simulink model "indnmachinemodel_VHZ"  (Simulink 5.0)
settings: Solver=ode4  StartTime=0  StopTime=1.2  FixedStep=1e-6  MaxStep=10e-6  RelTol=1e-3  AbsTol=1e-6
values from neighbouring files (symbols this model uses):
  J = 0.0226    [PARAM.M]
  p = 4    [PARAM.M]
  Rr = .39    (= 0.39)    [PARAM.M]
  Rs = .19    (= 0.19)    [PARAM.M]
  Vd = 300    [PARAM.M]
  wb = 2*pi*fb    (= 628.318530718)    [PARAM.M]
  Xlr = wb*Llr    (= 0.376991118431)    [PARAM.M]
  Xls = wb*Lls    (= 0.131946891451)    [PARAM.M]
  Xmstar = 1/(1/Xls+1/Xm+1/Xlr)    (= 0.0940797800005)    [PARAM.M]
undefined symbols (not defined in the file or in its folder): magnitude
libraries: simulink x2

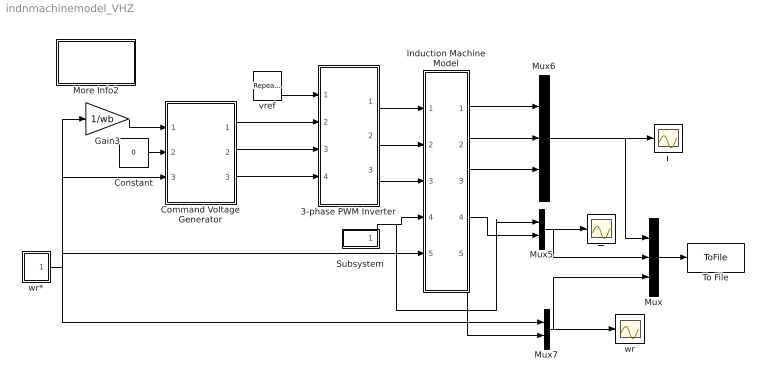
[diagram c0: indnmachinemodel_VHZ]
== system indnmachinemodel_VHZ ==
  3-phase PWM Inverter : Subsystem
  Command Voltage Generator : Subsystem
  Constant : Constant  Value=0
  Gain3 : Gain  Gain=1/wb
  Induction Machine Model : Subsystem
  More Info2 : Subsystem
  Mux : Mux  Inputs=3
  Mux5 : Mux  Inputs=2
  Mux6 : Mux  Inputs=3
  Mux7 : Mux  Inputs=2
  Subsystem : Subsystem
  T : Scope
  To File : ToFile  Filename=iemdc.mat  MatrixName=iemdc
  i : Scope
  vref : simulink/Sources/Repeating Sequence  rep_seq_t=[0 25e-6 50e-6 75e-6 100e-6]  rep_seq_y=[0 1 0 -1 0]
  wr : Scope
  wr* : Subsystem
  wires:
  Induction Machine Model/1(ia) -> Mux6/1
  Induction Machine Model/2(ib) -> Mux6/2
  Induction Machine Model/3(ic) -> Mux6/3
  Subsystem/1(Tl) -> Mux5/1, Induction Machine Model/4(Tl)
  Mux7/1 -> Mux/3, wr/1
  Mux5/1 -> Mux/2, T/1
  Induction Machine Model/4(Te) -> Mux5/2
  vref/1 -> 3-phase PWM Inverter/1(vref)
  wr*/1(wr*) -> Mux7/1, Induction Machine Model/5(we), Command Voltage Generator/3(we), Gain3/1
  Constant/1 -> Command Voltage Generator/2(vds*)
  Command Voltage Generator/1(vao*) -> 3-phase PWM Inverter/2(vao*)
  Command Voltage Generator/2(vbo*) -> 3-phase PWM Inverter/3(vbo*)
  Command Voltage Generator/3(vco*) -> 3-phase PWM Inverter/4(vco*)
  Induction Machine Model/5(wr) -> Mux7/2
  Gain3/1 -> Command Voltage Generator/1(vqs*)
  3-phase PWM Inverter/1(vao) -> Induction Machine Model/1(vao)
  3-phase PWM Inverter/2(vbo) -> Induction Machine Model/2(vbo)
  3-phase PWM Inverter/3(vco) -> Induction Machine Model/3(vco)
  Mux/1 -> To File/1
  Mux6/1 -> Mux/1, i/1

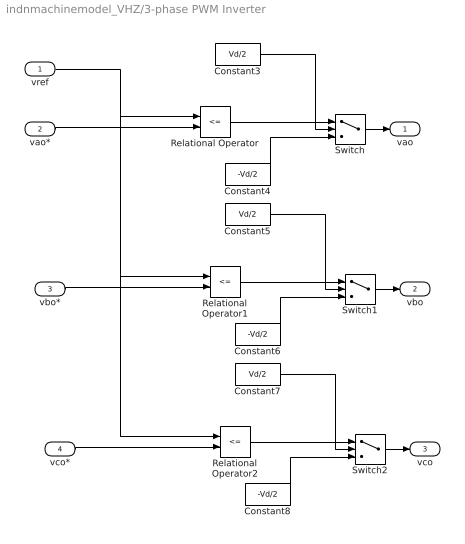
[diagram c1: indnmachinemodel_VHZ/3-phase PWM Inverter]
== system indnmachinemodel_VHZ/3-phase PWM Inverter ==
  vref : Inport
  vao* : Inport  Port=2
  vbo* : Inport  Port=3
  vco* : Inport  Port=4
  Constant3 : Constant  Value=Vd/2
  Constant4 : Constant  Value=-Vd/2
  Constant5 : Constant  Value=Vd/2
  Constant6 : Constant  Value=-Vd/2
  Constant7 : Constant  Value=Vd/2
  Constant8 : Constant  Value=-Vd/2
  Relational Operator : RelationalOperator  Operator=<=
  Relational Operator1 : RelationalOperator  Operator=<=
  Relational Operator2 : RelationalOperator  Operator=<=
  Switch : Switch  Threshold=0.5
  Switch1 : Switch  Threshold=0.5
  Switch2 : Switch  Threshold=0.5
  vao : Outport
  vbo : Outport  Port=2
  vco : Outport  Port=3
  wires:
  vao*/1 -> Relational Operator/2
  Switch/1 -> vao/1
  Constant4/1 -> Switch/3
  Constant3/1 -> Switch/1
  Relational Operator/1 -> Switch/2
  vbo*/1 -> Relational Operator1/2
  Switch1/1 -> vbo/1
  Constant6/1 -> Switch1/3
  Constant5/1 -> Switch1/1
  vco*/1 -> Relational Operator2/2
  Switch2/1 -> vco/1
  Constant8/1 -> Switch2/3
  Constant7/1 -> Switch2/1
  Relational Operator2/1 -> Switch2/2
  vref/1 -> Relational Operator/1, Relational Operator1/1, Relational Operator2/1
  Relational Operator1/1 -> Switch1/2

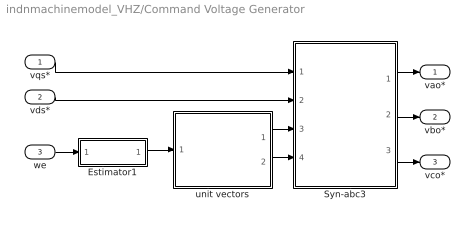
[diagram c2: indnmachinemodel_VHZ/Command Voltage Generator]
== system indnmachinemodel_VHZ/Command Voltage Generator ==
  vqs* : Inport
  vds* : Inport  Port=2
  we : Inport  Port=3
  Estimator1 : Subsystem
  Syn-abc3 : Subsystem
  unit vectors : Subsystem
  vao* : Outport
  vbo* : Outport  Port=2
  vco* : Outport  Port=3
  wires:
  Syn-abc3/1(vao*) -> vao*/1
  unit vectors/1(cos(theta-e)) -> Syn-abc3/3(cos(theta-e))
  unit vectors/2(sin(theta-e)) -> Syn-abc3/4(sin(theta-e))
  Estimator1/1(theta-e) -> unit vectors/1(theta-e)
  we/1 -> Estimator1/1(we)
  vds*/1 -> Syn-abc3/2(vds)
  vqs*/1 -> Syn-abc3/1(vqs)
  Syn-abc3/2(vbo*) -> vbo*/1
  Syn-abc3/3(vco*) -> vco*/1

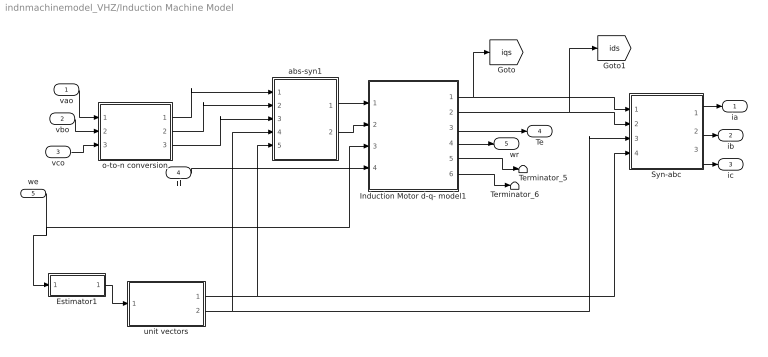
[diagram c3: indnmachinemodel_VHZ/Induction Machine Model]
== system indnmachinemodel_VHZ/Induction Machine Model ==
  vao : Inport
  vbo : Inport  Port=2
  vco : Inport  Port=3
  Tl : Inport  Port=4
  we : Inport  Port=5
  Estimator1 : Subsystem
  Induction Motor d-q- model1 : Subsystem
  Syn-abc : Subsystem
  Terminator_5 : Terminator
  Terminator_6 : Terminator
  abs-syn1 : Subsystem
  o-to-n conversion : Subsystem
  unit vectors : Subsystem
  ia : Outport
  ib : Outport  Port=2
  ic : Outport  Port=3
  Te : Outport  Port=4
  wr : Outport  Port=5
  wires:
  we/1 -> Induction Motor d-q- model1/3(we), Estimator1/1(we)
  Estimator1/1(theta-e) -> unit vectors/1(theta-e)
  Induction Motor d-q- model1/6("iqr ") -> Terminator_6/1
  Tl/1 -> Induction Motor d-q- model1/4(Tl)
  Syn-abc/2(ib) -> ib/1
  Syn-abc/3(ic) -> ic/1
  Induction Motor d-q- model1/5("idr ") -> Terminator_5/1
  Syn-abc/1(ia) -> ia/1
  Induction Motor d-q- model1/3("Te ") -> Te/1
  Induction Motor d-q- model1/4("wr ") -> wr/1
  vao/1 -> o-to-n conversion/1(vao)
  vbo/1 -> o-to-n conversion/2(vbo)
  vco/1 -> o-to-n conversion/3(vco)
  unit vectors/1(sin(theta-e)) -> Syn-abc/4(sin(theta-e)), abs-syn1/5(sin(theta-e))
  unit vectors/2(cos(theta-e)) -> Syn-abc/3(cos(theta-e)), abs-syn1/4(cos(theta-e))
  Induction Motor d-q- model1/2("ids ") -> Syn-abc/2(ids), [ids]
  Induction Motor d-q- model1/1("iqs ") -> [iqs], Syn-abc/1(iqs)
  o-to-n conversion/1(van) -> abs-syn1/1(van)
  o-to-n conversion/2(vbn) -> abs-syn1/2(vbn)
  o-to-n conversion/3(vcn) -> abs-syn1/3(vcn)
  abs-syn1/2(vds) -> Induction Motor d-q- model1/2(vds)
  abs-syn1/1(vqs) -> Induction Motor d-q- model1/1(vqs)

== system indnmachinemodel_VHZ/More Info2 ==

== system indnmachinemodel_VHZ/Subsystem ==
  Step2 : Step  Time=.8  After=20  SampleTime=0
  Step3 : Step  After=-10  SampleTime=0
  Step4 : Step  Time=30  After=0  SampleTime=0
  Sum1 : Sum  Inputs=|+++
  Tl : Outport
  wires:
  Step3/1 -> Sum1/2
  Step2/1 -> Sum1/1
  Step4/1 -> Sum1/3
  Sum1/1 -> Tl/1

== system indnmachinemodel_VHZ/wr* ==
  Gain2 : Gain
  Repeating Sequence : simulink/Sources/Repeating Sequence  rep_seq_t=[0 .15 .35 .4 .55 .6 10]  rep_seq_y=[0 .8*wb .8*wb .50*wb .50*wb .65*wb .65*wb]
  Saturation1 : Saturate  UpperLimit=.75*wb  LowerLimit=-.75*wb
  wr* : Outport
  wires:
  Repeating Sequence/1 -> Saturation1/1
  Saturation1/1 -> Gain2/1
  Gain2/1 -> wr*/1

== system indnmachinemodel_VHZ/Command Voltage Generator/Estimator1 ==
  we : Inport
  Constant : Constant  Value=2*pi
  Integrator : Integrator
  Math Function3 : Math  Operator=mod
  theta-e : Outport
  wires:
  Math Function3/1 -> theta-e/1
  Integrator/1 -> Math Function3/1
  Constant/1 -> Math Function3/2
  we/1 -> Integrator/1

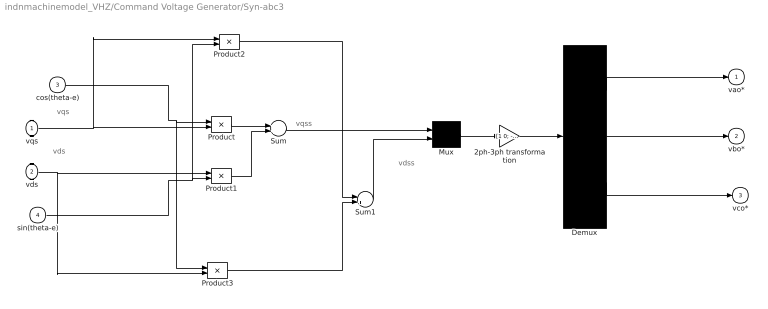
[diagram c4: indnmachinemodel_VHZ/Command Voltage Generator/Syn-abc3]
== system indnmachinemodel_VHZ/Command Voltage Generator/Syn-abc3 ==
  note: vqss
  note: vqs
  note: vdss
  note: vds
  vqs : Inport
  vds : Inport  Port=2
  cos(theta-e) : Inport  Port=3
  sin(theta-e) : Inport  Port=4
  2ph-3ph transformation : Gain  Gain="[1 0; -1/2 -sqrt(3)/2;  -1/2 sqrt(3)/2]"  Multiplication=Matrix(K*u)
  Demux : Demux  Outputs=3
  Mux : Mux  Inputs=2
  Product{,1..3} (4 alike) : Product
  Sum : Sum
  Sum1 : Sum  Inputs=-+
  vao* : Outport
  vbo* : Outport  Port=2
  vco* : Outport  Port=3
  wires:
  2ph-3ph transformation/1 -> Demux/1
  Sum1/1 -> Mux/2
  Product/1 -> Sum/1
  Product1/1 -> Sum/2
  sin(theta-e)/1 -> Product2/2, Product1/2
  cos(theta-e)/1 -> Product3/1, Product/1
  Product3/1 -> Sum1/2
  Product2/1 -> Sum1/1
  Mux/1 -> 2ph-3ph transformation/1
  vds/1 -> Product3/2, Product1/1
  vqs/1 -> Product2/1, Product/2
  Demux/1 -> vao*/1
  Demux/2 -> vbo*/1
  Demux/3 -> vco*/1
  Sum/1 -> Mux/1

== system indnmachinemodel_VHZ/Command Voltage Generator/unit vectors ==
  theta-e : Inport
  Trigonometric Function : Trigonometry
  Trigonometric Function1 : Trigonometry  Operator=cos
  cos(theta-e) : Outport
  sin(theta-e) : Outport  Port=2
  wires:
  Trigonometric Function/1 -> sin(theta-e)/1
  Trigonometric Function1/1 -> cos(theta-e)/1
  theta-e/1 -> Trigonometric Function1/1, Trigonometric Function/1

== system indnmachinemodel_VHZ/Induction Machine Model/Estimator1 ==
  we : Inport
  Constant : Constant  Value=2*pi
  Integrator : Integrator  InitialCondition=0.01
  Math Function3 : Math  Operator=mod
  theta-e : Outport
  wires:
  we/1 -> Integrator/1
  Constant/1 -> Math Function3/2
  Integrator/1 -> Math Function3/1
  Math Function3/1 -> theta-e/1

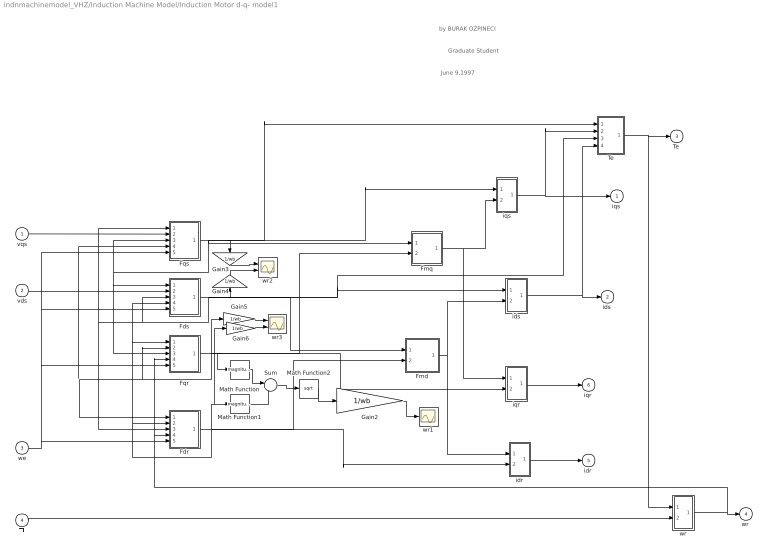
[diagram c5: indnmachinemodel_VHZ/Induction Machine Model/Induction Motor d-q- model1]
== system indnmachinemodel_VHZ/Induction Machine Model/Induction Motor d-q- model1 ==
  note: by BURAK OZPINECI
  note: Graduate Student
  note: June 9,1997
  vqs : Inport
  vds : Inport  Port=2
  we : Inport  Port=3
  Tl : Inport  Port=4
  Fdr : Subsystem
  Fds : Subsystem
  Fmd : Subsystem
  Fmq : Subsystem
  Fqr : Subsystem
  Fqs : Subsystem
  Gain2 : Gain  Gain=1/wb
  Gain3 : Gain  Orientation=down  Gain=1/wb
  Gain4 : Gain  Orientation=up  Gain=1/wb
  Gain5 : Gain  Gain=1/wb
  Gain6 : Gain  Gain=1/wb
  Math Function : Math  Operator=magnitude^2
  Math Function1 : Math  Operator=magnitude^2
  Math Function2 : Math  Operator=sqrt
  Sum : Sum  Inputs=|++
  Te : Subsystem
  idr : Subsystem
  ids : Subsystem
  iqr : Subsystem
  iqs : Subsystem
  wr : Subsystem
  wr1 : Scope
  wr2 : Scope  NumInputPorts=2
  wr3 : Scope  NumInputPorts=2
  "iqs " : Outport
  "ids " : Outport  Port=2
  "Te " : Outport  Port=3
  "wr " : Outport  Port=4
  "idr " : Outport  Port=5
  "iqr " : Outport  Port=6
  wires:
  Fdr/1("Fdr ") -> idr/2(Fdr), Fdr/2(Fdr), Fqr/1(Fdr), Fds/4(Fdr), Fmd/2(Fdr), Math Function1/1, Gain6/1
  we/1 -> Fqs/5(we), Fds/5(we), Fqr/5(we), Fdr/5(we)
  wr/1(wr) -> "wr "/1, Fqr/4(wr), Fdr/4(wr)
  vqs/1 -> Fqs/2(Vqs)
  vds/1 -> Fds/2(Vds)
  Tl/1 -> wr/2(Tl)
  Fqs/1("Fqs ") -> Fqs/3(Fqs), Fqr/3(Fqs), Fds/1(Fqs), Fmq/1(Fqs), iqs/1(Fqs), Te/1(Fqs), Gain3/1
  Fqr/1("Fqr ") -> Fqr/2(Fqr), Fqs/4(Fqr), Fdr/1(Fqr), Fmq/2(Fqr), Math Function/1, iqr/2(Fqr), Gain5/1
  Fds/1("Fds ") -> Fds/3(Fds), Fqs/1(Fds), Fdr/3(Fds), Fmd/1(Fds), ids/1(Fds), Te/3(Fds), Gain4/1
  iqr/1(iqr) -> "iqr "/1
  Fmq/1(Fmq) -> iqs/2(Fmq), iqr/1(Fmq)
  idr/1(idr) -> "idr "/1
  Fmd/1(Fmd) -> ids/2(Fmd), idr/1(Fmd)
  Te/1(Te) -> "Te "/1, wr/1(Te)
  ids/1(ids) -> "ids "/1, Te/4(ids)
  iqs/1(iqs) -> "iqs "/1, Te/2(iqs)
  Math Function/1 -> Sum/1
  Math Function1/1 -> Sum/2
  Sum/1 -> Math Function2/1
  Math Function2/1 -> Gain2/1
  Gain2/1 -> wr1/1
  Gain3/1 -> wr2/1
  Gain4/1 -> wr2/2
  Gain5/1 -> wr3/1
  Gain6/1 -> wr3/2

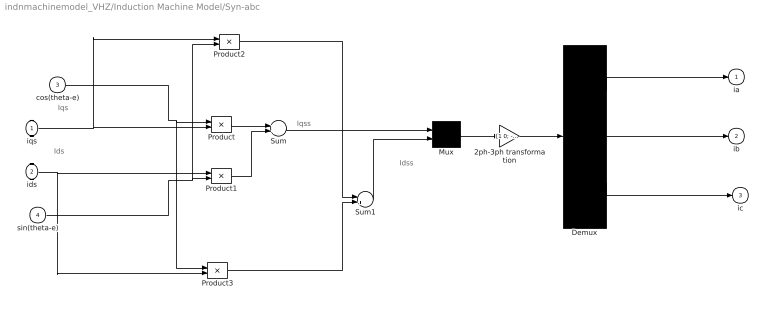
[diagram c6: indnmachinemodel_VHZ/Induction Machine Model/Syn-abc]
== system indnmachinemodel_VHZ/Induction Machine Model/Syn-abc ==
  note: Iqss
  note: Iqs
  note: Idss
  note: Ids
  iqs : Inport
  ids : Inport  Port=2
  cos(theta-e) : Inport  Port=3
  sin(theta-e) : Inport  Port=4
  2ph-3ph transformation : Gain  Gain="[1 0; -1/2 -sqrt(3)/2;  -1/2 sqrt(3)/2]"  Multiplication=Matrix(K*u)
  Demux : Demux  Outputs=3
  Mux : Mux  Inputs=2
  Product{,1..3} (4 alike) : Product
  Sum : Sum
  Sum1 : Sum  Inputs=-+
  ia : Outport
  ib : Outport  Port=2
  ic : Outport  Port=3
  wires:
  2ph-3ph transformation/1 -> Demux/1
  Sum1/1 -> Mux/2
  Sum/1 -> Mux/1
  Product/1 -> Sum/1
  Product1/1 -> Sum/2
  sin(theta-e)/1 -> Product2/2, Product1/2
  cos(theta-e)/1 -> Product3/1, Product/1
  Product3/1 -> Sum1/2
  Product2/1 -> Sum1/1
  Mux/1 -> 2ph-3ph transformation/1
  ids/1 -> Product3/2, Product1/1
  iqs/1 -> Product2/1, Product/2
  Demux/1 -> ia/1
  Demux/2 -> ib/1
  Demux/3 -> ic/1

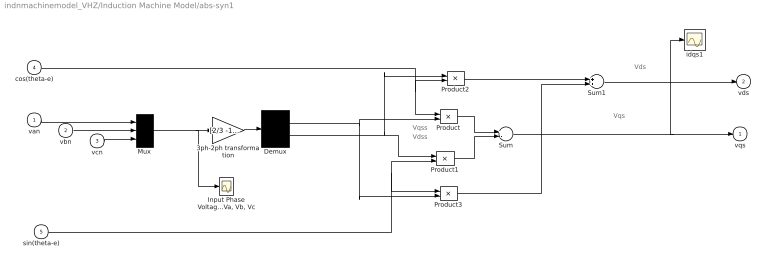
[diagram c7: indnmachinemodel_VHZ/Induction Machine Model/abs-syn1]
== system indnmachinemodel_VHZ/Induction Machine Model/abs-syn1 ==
  note: Vqs
  note: Vds
  note: Vqss
  note: Vdss
  van : Inport
  vbn : Inport  Port=2
  vcn : Inport  Port=3
  cos(theta-e) : Inport  Port=4
  sin(theta-e) : Inport  Port=5
  3ph-2ph transformation : Gain  Gain=[2/3 -1/3 -1/3;0 -1/sqrt(3) 1/sqrt(3)]  Multiplication=Matrix(K*u)
  Demux : Demux  Outputs=2
  "Input Phase Voltages Va, Vb, Vc" : Scope
  Mux : Mux  Inputs=3
  Product{,1..3} (4 alike) : Product
  Sum : Sum  Inputs=+-
  Sum1 : Sum
  idqs1 : Scope
  vqs : Outport
  vds : Outport  Port=2
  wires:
  cos(theta-e)/1 -> Product2/2, Product/1
  sin(theta-e)/1 -> Product3/1, Product1/2
  Demux/1 -> Product3/2, Product/2
  van/1 -> Mux/1
  Demux/2 -> Product1/1, Product2/1
  vbn/1 -> Mux/2
  Product3/1 -> Sum1/2
  Product2/1 -> Sum1/1
  Sum/1 -> idqs1/1, vqs/1
  Sum1/1 -> vds/1
  Product1/1 -> Sum/2
  Mux/1 -> 3ph-2ph transformation/1, "Input Phase Voltages Va, Vb, Vc"/1
  vcn/1 -> Mux/3
  Product/1 -> Sum/1
  3ph-2ph transformation/1 -> Demux/1

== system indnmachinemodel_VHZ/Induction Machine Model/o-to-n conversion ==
  vao : Inport
  vbo : Inport  Port=2
  vco : Inport  Port=3
  Demux : Demux  Outputs=3
  Matrix Gain : Gain  Gain=[2/3 -1/3 -1/3; -1/3 2/3 -1/3; -1/3 -1/3 2/3]  Multiplication=Matrix(K*u)
  Mux : Mux  Inputs=3
  van : Outport
  vbn : Outport  Port=2
  vcn : Outport  Port=3
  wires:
  Demux/3 -> vcn/1
  Demux/2 -> vbn/1
  Demux/1 -> van/1
  vco/1 -> Mux/3
  vbo/1 -> Mux/2
  vao/1 -> Mux/1
  Matrix Gain/1 -> Demux/1
  Mux/1 -> Matrix Gain/1

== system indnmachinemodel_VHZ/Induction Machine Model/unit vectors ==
  theta-e : Inport
  Trigonometric Function : Trigonometry
  Trigonometric Function1 : Trigonometry  Operator=cos
  sin(theta-e) : Outport
  cos(theta-e) : Outport  Port=2
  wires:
  theta-e/1 -> Trigonometric Function/1, Trigonometric Function1/1
  Trigonometric Function1/1 -> cos(theta-e)/1
  Trigonometric Function/1 -> sin(theta-e)/1

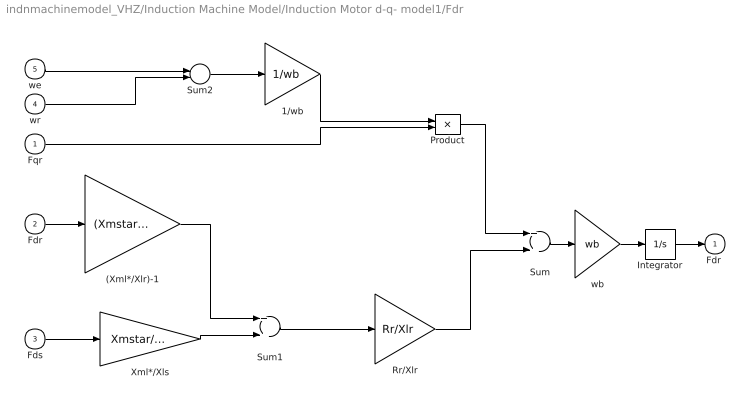
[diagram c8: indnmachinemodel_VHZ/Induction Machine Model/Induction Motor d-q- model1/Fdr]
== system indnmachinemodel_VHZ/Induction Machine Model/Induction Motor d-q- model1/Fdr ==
  Fqr : Inport
  Fdr : Inport  Port=2
  Fds : Inport  Port=3
  wr : Inport  Port=4
  we : Inport  Port=5
  (Xml*/Xlr)-1 : Gain  Gain=(Xmstar/Xlr)-1
  1/wb : Gain  Gain=1/wb
  Integrator : Integrator
  Product : Product
  Rr/Xlr : Gain  Gain=Rr/Xlr
  Sum : Sum
  Sum1 : Sum
  Sum2 : Sum  Inputs=+-
  Xml*/Xls : Gain  Gain=Xmstar/Xls
  wb : Gain  Gain=wb
  "Fdr " : Outport
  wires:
  Rr/Xlr/1 -> Sum/2
  Xml*/Xls/1 -> Sum1/2
  (Xml*/Xlr)-1/1 -> Sum1/1
  Product/1 -> Sum/1
  1/wb/1 -> Product/1
  wr/1 -> Sum2/2
  Fqr/1 -> Product/2
  we/1 -> Sum2/1
  Sum2/1 -> 1/wb/1
  Fds/1 -> Xml*/Xls/1
  Integrator/1 -> "Fdr "/1
  Fdr/1 -> (Xml*/Xlr)-1/1
  Sum1/1 -> Rr/Xlr/1
  Sum/1 -> wb/1
  wb/1 -> Integrator/1

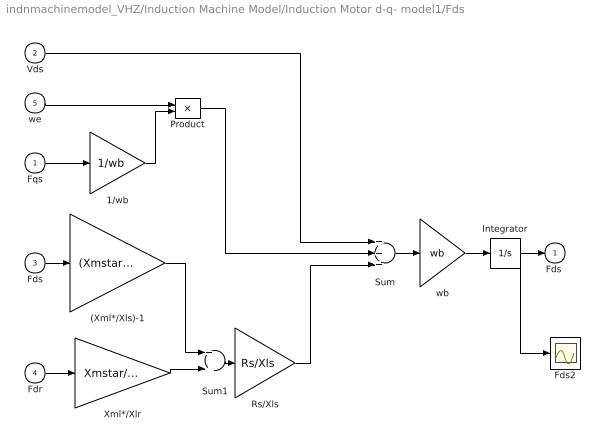
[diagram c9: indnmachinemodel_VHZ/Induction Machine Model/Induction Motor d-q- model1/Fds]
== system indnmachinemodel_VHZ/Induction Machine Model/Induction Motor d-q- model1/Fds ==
  Fqs : Inport
  Vds : Inport  Port=2
  Fds : Inport  Port=3
  Fdr : Inport  Port=4
  we : Inport  Port=5
  (Xml*/Xls)-1 : Gain  Gain=(Xmstar/Xls)-1
  1/wb : Gain  Gain=1/wb
  Fds2 : Scope
  Integrator : Integrator
  Product : Product
  Rs/Xls : Gain  Gain=Rs/Xls
  Sum : Sum  Inputs=+++
  Sum1 : Sum
  Xml*/Xlr : Gain  Gain=Xmstar/Xlr
  wb : Gain  Gain=wb
  "Fds " : Outport
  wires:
  1/wb/1 -> Product/2
  Product/1 -> Sum/2
  we/1 -> Product/1
  wb/1 -> Integrator/1
  Fdr/1 -> Xml*/Xlr/1
  Fds/1 -> (Xml*/Xls)-1/1
  Vds/1 -> Sum/1
  Fqs/1 -> 1/wb/1
  Rs/Xls/1 -> Sum/3
  (Xml*/Xls)-1/1 -> Sum1/1
  Xml*/Xlr/1 -> Sum1/2
  Sum1/1 -> Rs/Xls/1
  Sum/1 -> wb/1
  Integrator/1 -> "Fds "/1, Fds2/1

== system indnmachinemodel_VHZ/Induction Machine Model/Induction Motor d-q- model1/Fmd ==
  Fds : Inport
  Fdr : Inport  Port=2
  Sum8 : Sum
  Xmstar/Xlr : Gain  Gain=Xmstar/Xlr
  Xmstar/Xls : Gain  Gain=Xmstar/Xls
  Fmd : Outport
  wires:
  Fdr/1 -> Xmstar/Xlr/1
  Sum8/1 -> Fmd/1
  Fds/1 -> Xmstar/Xls/1
  Xmstar/Xls/1 -> Sum8/1
  Xmstar/Xlr/1 -> Sum8/2

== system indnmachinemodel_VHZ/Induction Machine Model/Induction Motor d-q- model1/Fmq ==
  Fqs : Inport
  Fqr : Inport  Port=2
  Sum8 : Sum
  Xmstar/Xlr : Gain  Gain=Xmstar/Xlr
  Xmstar/Xls : Gain  Gain=Xmstar/Xls
  Fmq : Outport
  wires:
  Fqr/1 -> Xmstar/Xlr/1
  Sum8/1 -> Fmq/1
  Fqs/1 -> Xmstar/Xls/1
  Xmstar/Xls/1 -> Sum8/1
  Xmstar/Xlr/1 -> Sum8/2

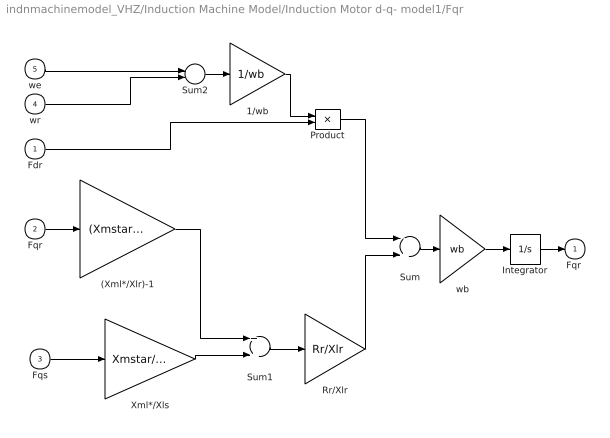
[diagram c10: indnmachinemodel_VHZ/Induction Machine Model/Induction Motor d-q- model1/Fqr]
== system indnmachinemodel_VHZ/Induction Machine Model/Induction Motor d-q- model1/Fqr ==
  Fdr : Inport
  Fqr : Inport  Port=2
  Fqs : Inport  Port=3
  wr : Inport  Port=4
  we : Inport  Port=5
  (Xml*/Xlr)-1 : Gain  Gain=(Xmstar/Xlr)-1
  1/wb : Gain  Gain=1/wb
  Integrator : Integrator
  Product : Product
  Rr/Xlr : Gain  Gain=Rr/Xlr
  Sum : Sum  Inputs=-+
  Sum1 : Sum
  Sum2 : Sum  Inputs=+-
  Xml*/Xls : Gain  Gain=Xmstar/Xls
  wb : Gain  Gain=wb
  "Fqr " : Outport
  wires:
  (Xml*/Xlr)-1/1 -> Sum1/1
  Rr/Xlr/1 -> Sum/2
  Product/1 -> Sum/1
  Fdr/1 -> Product/2
  1/wb/1 -> Product/1
  Sum2/1 -> 1/wb/1
  wr/1 -> Sum2/2
  we/1 -> Sum2/1
  Fqs/1 -> Xml*/Xls/1
  Integrator/1 -> "Fqr "/1
  Fqr/1 -> (Xml*/Xlr)-1/1
  Xml*/Xls/1 -> Sum1/2
  Sum1/1 -> Rr/Xlr/1
  Sum/1 -> wb/1
  wb/1 -> Integrator/1

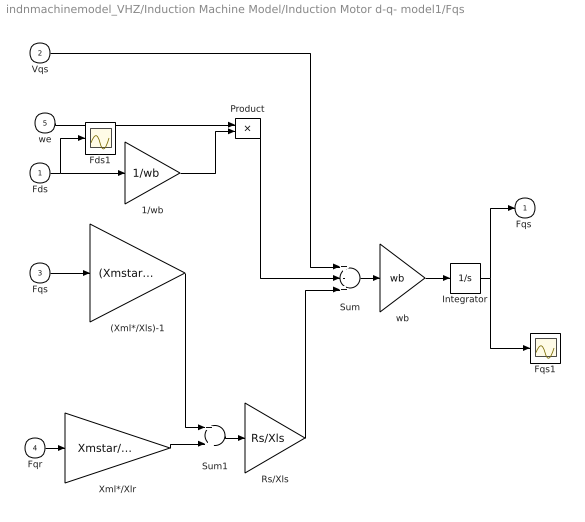
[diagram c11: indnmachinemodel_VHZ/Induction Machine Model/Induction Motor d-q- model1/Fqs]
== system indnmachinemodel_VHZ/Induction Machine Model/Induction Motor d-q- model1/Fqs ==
  Fds : Inport
  Vqs : Inport  Port=2
  Fqs : Inport  Port=3
  Fqr : Inport  Port=4
  we : Inport  Port=5
  (Xml*/Xls)-1 : Gain  Gain=(Xmstar/Xls)-1
  1/wb : Gain  Gain=1/wb
  Fds1 : Scope
  Fqs1 : Scope
  Integrator : Integrator
  Product : Product
  Rs/Xls : Gain  Gain=Rs/Xls
  Sum : Sum  Inputs=+-+
  Sum1 : Sum
  Xml*/Xlr : Gain  Gain=Xmstar/Xlr
  wb : Gain  Gain=wb
  "Fqs " : Outport
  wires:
  1/wb/1 -> Product/2
  Product/1 -> Sum/2
  we/1 -> Product/1
  Xml*/Xlr/1 -> Sum1/2
  (Xml*/Xls)-1/1 -> Sum1/1
  wb/1 -> Integrator/1
  Fqr/1 -> Xml*/Xlr/1
  Fqs/1 -> (Xml*/Xls)-1/1
  Vqs/1 -> Sum/1
  Rs/Xls/1 -> Sum/3
  Sum1/1 -> Rs/Xls/1
  Sum/1 -> wb/1
  Integrator/1 -> "Fqs "/1, Fqs1/1
  Fds/1 -> 1/wb/1, Fds1/1

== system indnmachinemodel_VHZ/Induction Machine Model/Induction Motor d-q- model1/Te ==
  Fqs : Inport
  iqs : Inport  Port=2
  Fds : Inport  Port=3
  ids : Inport  Port=4
  3*p/(4*wb) : Gain  Gain=3*p/(4*wb)
  Product : Product
  Product1 : Product
  Sum7 : Sum  Inputs=+-
  Te : Outport
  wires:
  ids/1 -> Product/2
  Fqs/1 -> Product/1
  iqs/1 -> Product1/2
  Fds/1 -> Product1/1
  3*p/(4*wb)/1 -> Te/1
  Sum7/1 -> 3*p/(4*wb)/1
  Product1/1 -> Sum7/1
  Product/1 -> Sum7/2

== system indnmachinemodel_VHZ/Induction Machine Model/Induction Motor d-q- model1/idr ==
  Fmd : Inport
  Fdr : Inport  Port=2
  1/Xlr : Gain  Gain=1/Xlr
  Sum8 : Sum  Inputs=+-
  idr : Outport
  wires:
  Fmd/1 -> Sum8/2
  1/Xlr/1 -> idr/1
  Fdr/1 -> Sum8/1
  Sum8/1 -> 1/Xlr/1

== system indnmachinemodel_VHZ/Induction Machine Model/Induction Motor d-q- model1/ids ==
  Fds : Inport
  Fmd : Inport  Port=2
  1/Xls : Gain  Gain=1/Xls
  Sum8 : Sum  Inputs=+-
  ids : Outport
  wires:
  Fmd/1 -> Sum8/2
  1/Xls/1 -> ids/1
  Fds/1 -> Sum8/1
  Sum8/1 -> 1/Xls/1

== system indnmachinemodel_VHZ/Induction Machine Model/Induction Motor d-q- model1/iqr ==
  Fmq : Inport
  Fqr : Inport  Port=2
  1/Xlr : Gain  Gain=1/Xlr
  Sum8 : Sum  Inputs=+-
  iqr : Outport
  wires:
  Fmq/1 -> Sum8/2
  1/Xlr/1 -> iqr/1
  Fqr/1 -> Sum8/1
  Sum8/1 -> 1/Xlr/1

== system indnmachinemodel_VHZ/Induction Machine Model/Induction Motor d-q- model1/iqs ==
  Fqs : Inport
  Fmq : Inport  Port=2
  1/Xls : Gain  Gain=1/Xls
  Sum8 : Sum  Inputs=+-
  iqs : Outport
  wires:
  Fmq/1 -> Sum8/2
  1/Xls/1 -> iqs/1
  Fqs/1 -> Sum8/1
  Sum8/1 -> 1/Xls/1

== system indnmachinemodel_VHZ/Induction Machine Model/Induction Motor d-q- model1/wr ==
  Te : Inport
  Tl : Inport  Port=2
  Integrator : Integrator
  Sum7 : Sum  Inputs=+-
  p/(2*J) : Gain  Gain=p/(2*J)
  wr : Outport
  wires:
  Te/1 -> Sum7/1
  Tl/1 -> Sum7/2
  Integrator/1 -> wr/1
  p/(2*J)/1 -> Integrator/1
  Sum7/1 -> p/(2*J)/1
